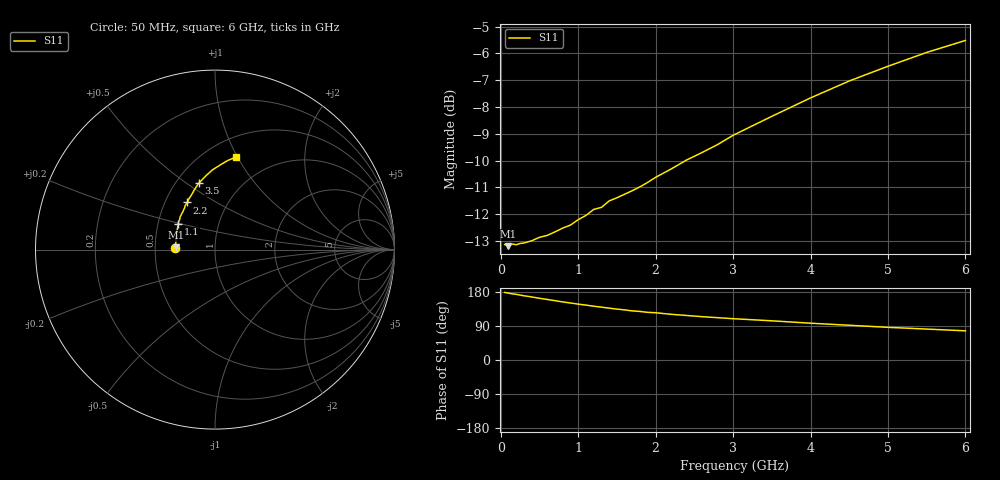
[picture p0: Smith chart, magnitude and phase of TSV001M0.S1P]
! SIEMENS Small Signal Semiconductors
! BAT14-03W
! Si Schottky Diode in SOD323
! IF = 1 mA
! S-Parameters:  November  1995
# GHz  S  MA  R  50
!  f  S11
! GHz  MAG  ANG
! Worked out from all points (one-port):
!   34 points, 50 MHz to 6 GHz, reference 50 ohm
!   lowest |S11| = -13.2 dB at 100 MHz (marker M1), VSWR 1.56, Z = 32 + j0.926 ohm
!   |S11| at or under -10 dB: start of sweep to 2.385 GHz
!   S11 on the Smith chart (normalised r, x): 50 MHz: 0.64, +0.01; 1.1 GHz: 0.64, +0.20; 2.2 GHz: 0.65, +0.37; 3.5 GHz: 0.65, +0.56; 6 GHz: 0.69, +0.99
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0.05  0.2207 178.4
0.1  0.2191 176.4
0.15  0.2212 174.6
0.2  0.2205 173.3
0.4  0.2243 166.4
0.5  0.2276 162.8
0.6  0.2295 159.8
0.8  0.2368 153.2
0.9  0.2399 150.4
1.1  0.25 144.9
1.2  0.2565 141.9
1.3  0.2588 139.5
1.4  0.2661 136.9
1.6  0.2738 132.2
1.7  0.2781 129.6
1.8  0.2828 128.1
1.9  0.2882 125.7
2  0.2944 124.7
2.2  0.3051 120.6
2.4  0.3171 117.5
2.8  0.3388 111.7
3  0.3526 109.0
3.5  0.3825 103.4
4  0.4139 97.1
4.5  0.4451 91.7
5  0.4741 86.2
5.5  0.5031 81.6
6  0.5297 77.0
